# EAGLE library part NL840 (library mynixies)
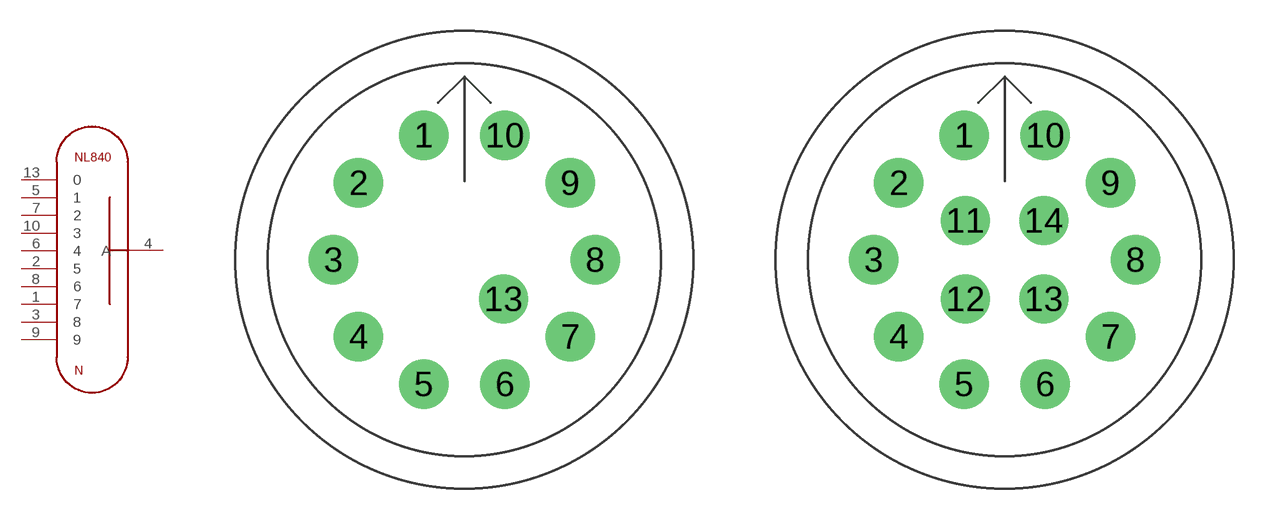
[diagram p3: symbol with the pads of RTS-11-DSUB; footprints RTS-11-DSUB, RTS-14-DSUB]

Designator prefix N

## NL840RTS-11  [RTS-11-DSUB]
1  7  pas
2  5  pas
3  8  pas
4  A  pas
5  1  pas
6  4  pas
7  2  pas
8  6  pas
9  9  pas
10  3  pas
13  0  pas

## NL840RTS-14  [RTS-14-DSUB]
Pads as for RTS-11-DSUB

## Footprint RTS-11-DSUB (pad centres in mm)
drill 1.6: 1 -1.962,6.039; 2 -5.137,3.732; 3 -6.35,0; 4 -5.137,-3.732; 5 -1.962,-6.039; 6 1.962,-6.039; 7 5.137,-3.732; 8 6.35,0; 9 5.137,3.732; 10 1.962,6.039; 13 1.904,-1.904

## Footprint RTS-14-DSUB (pad centres in mm)
drill 1.6: 1 -1.962,6.039; 2 -5.137,3.732; 3 -6.35,0; 4 -5.137,-3.732; 5 -1.962,-6.039; 6 1.962,-6.039; 7 5.137,-3.732; 8 6.35,0; 9 5.137,3.732; 10 1.962,6.039; 11 -1.904,1.904; 12 -1.904,-1.904; 13 1.904,-1.904; 14 1.904,1.904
